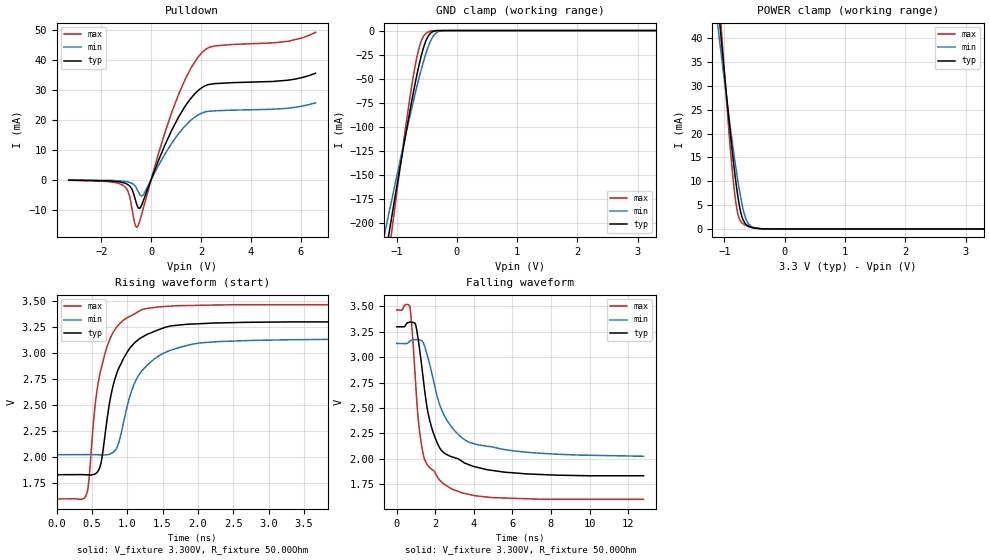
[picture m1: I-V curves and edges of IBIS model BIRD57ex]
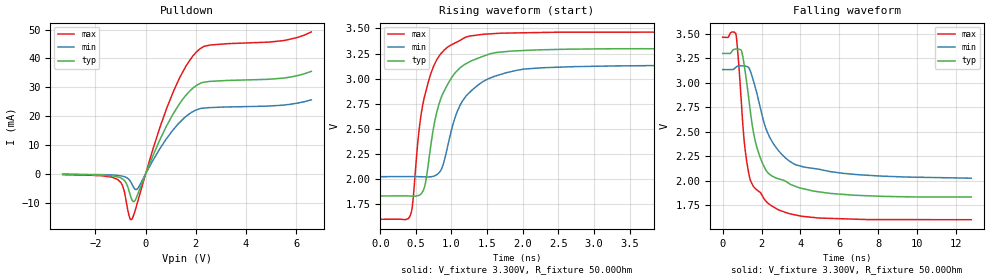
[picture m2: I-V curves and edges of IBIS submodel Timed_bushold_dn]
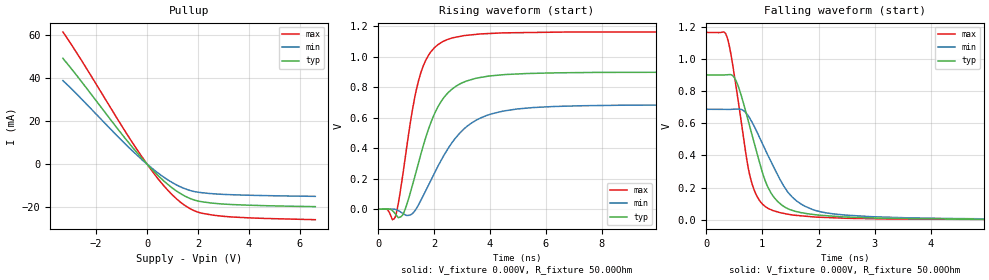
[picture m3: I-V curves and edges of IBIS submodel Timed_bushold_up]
[IBIS Ver]   3.2
[File name]   bird57ex.ibs
[File rev]   0.00
[Date]   12/9/98
[Source]   From silicon level BOGUS SPICE model.
[Notes]   The following information uses the features of BIRD57 to
   describe a FICTICIOUS chip which has an active termintor.
[Disclaimer] This information is only for demonstrating how BIRD57
   works and does not represent any real device in production
   or design.
   WARNING: THIS MODEL HAS NOT BEEN CHECKED USING IBISCHK3.2
   WHICH IS UNDER DEVELOPMENT.  IT MAY CONTAIN SYNTAX ERRORS.
[Copyright]   None - public sample
[Component]   BIRD57ex
[Manufacturer]  Nobody
[Package]
|   typ   min   max
R_pkg   100.00mOhm   NA   NA
L_pkg   8.00nH   NA   NA
C_pkg   5.00pF   NA   NA
[Pin]   signal_name   model_name   R_pin   L_pin   C_pin
1   Vcc   POWER
2   GND   GND
3   Data   BIRD57ex
| Models and submodels in the file (3): BIRD57ex (I/O_open_sink), Timed_bushold_dn (Bus_hold), Timed_bushold_up (Bus_hold)
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[Model]   BIRD57ex
Model_type   I/O_open_sink
Vinl = 800.00mV
Vinh = 2.00V
Vmeas = 1.50V
Cref = 0.00F
|   typ   min   max
C_comp   4.00pF   2.00pF   6.00pF
[Voltage Range]   3.300V   3.135V   3.465V
[Temperature Range]   50.0   100.0   0.0
[Add Submodel]
| name   mode
Timed_bushold_up   All
Timed_bushold_dn   Non-Driving
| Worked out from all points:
|   slope of the pulldown table from 0 to 0.495 V, typ, clamps not added: 47.7 ohm
|   GND clamp passes 1 mA (typ) near -0.39 V on its own axis
|   POWER clamp passes 1 mA (typ) near -0.64 V on its own axis
|   falling waveform, V_fixture 3.300V, R_fixture 50.00Ohm: 20-80 % time 941ps typ, 1.42ns min, 633ps max; typ from 3.3 V to 1.83 V
|   rising waveform, V_fixture 3.300V, R_fixture 50.00Ohm: 20-80 % time 328ps typ, 412ps min, 250ps max; typ from 1.83 V to 3.3 V
[Pulldown]
|   Voltage   I(typ)   I(min)   I(max)
-3.3V     -135.8uA   -78.2uA    -215.1uA
-1.025V   -1.197mA   NA         NA
-785mV    -2.945mA   -1.129mA   NA
-705mV    -4.542mA   NA         NA
-555mV    -8.746mA   NA         NA
-365mV    -8.224mA   NA         NA
825mV     16.45mA    NA         NA
1.46V     25.65mA    NA         NA
2.055V    30.81mA    NA         NA
2.56V     32.06mA    NA         NA
5.47V     33.18mA    NA         NA
6.6V      35.53mA    25.66mA    49.18mA
[GND Clamp]
|   Voltage   I(typ)   I(min)   I(max)
-3.3V     -1.1A      -859.8mA   -1.35A
-1.265V   -264.8mA   NA         -300.4mA
-1.135V   -214.8mA   NA         -235.9mA
-1.075V   -191.9mA   NA         NA
-825mV    -99.88mA   NA         NA
-690mV    -54.59mA   NA         NA
-585mV    -25.13mA   -39.38mA   NA
-520mV    -11.92mA   -25.29mA   NA
-460mV    -4.469mA   NA         NA
-370mV    -529.2uA   NA         NA
-285mV    -44.47uA   NA         NA
3.3V      0A         0A         0A
[POWER Clamp]
|   Voltage   I(typ)   I(min)   I(max)
-3.3V     370mA      287.5mA    500mA
-1.145V   52.63mA    46.39mA    NA
-1.095V   45.64mA    41.06mA    NA
-1.045V   38.76mA    35.79mA    NA
-895mV    19.25mA    NA         15.81mA
-820mV    10.8mA     13.69mA    NA
-775mV    6.621mA    NA         NA
-735mV    3.82mA     NA         NA
-655mV    1.132mA    2.538mA    NA
-575mV    429.4uA    NA         NA
-365mV    19.18uA    NA         NA
3.3V      0A         0A         0A
[Ramp]
R_load = 50.00Ohm
|   typ   min   max
dV/dt_r   540.04mV/1.04ns   411.75mV/1.47ns   698.42mV/705.58ps
dV/dt_f   879.96mV/936.61ps   666.10mV/1.42ns   1.12V/623.48ps
[Falling Waveform]
V_fixture = 3.300V
V_fixture_min = 3.135V
V_fixture_max = 3.465V
R_fixture = 50.00Ohm
|   Time   V(typ)   V(min)   V(max)
0s        3.3V       3.135V     3.465V
670ps     3.346V     NA         NA
970ps     3.324V     NA         NA
1.18ns    3.084V     NA         NA
1.45ns    2.666V     NA         NA
1.78ns    2.326V     NA         NA
2.42ns    2.063V     NA         NA
3.18ns    2.001V     NA         NA
3.96ns    1.926V     NA         NA
12.8ns    1.833V     2.025V     1.601V
[Rising Waveform]
V_fixture = 3.300V
V_fixture_min = 3.135V
V_fixture_max = 3.465V
R_fixture = 50.00Ohm
|   Time   V(typ)   V(min)   V(max)
0s        1.833V     2.025V     1.601V
370ps     1.834V     NA         NA
490ps     1.83V      NA         NA
580ps     1.86V      NA         NA
710ps     2.339V     NA         NA
850ps     2.802V     NA         NA
1.05ns    3.058V     NA         NA
1.28ns    3.178V     NA         NA
2.67ns    3.294V     NA         NA
12.8ns    3.3V       3.135V     3.465V
[Submodel]   Timed_bushold_dn
Submodel_type   Bus_hold
[Submodel Spec]
|   typ   min   max
V_trigger_r   15.00   15.00   15.00
V_trigger_f   1.65   1.50   1.80
Off_delay   5.00ns   3.00ns   7.00ns
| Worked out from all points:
|   slope of the pulldown table from 0 to 0.3 V, typ, clamps not added: 46.2 ohm
|   falling waveform, V_fixture 3.300V, R_fixture 50.00Ohm: 20-80 % time 941ps typ, 1.42ns min, 633ps max; typ from 3.3 V to 1.83 V
|   rising waveform, V_fixture 3.300V, R_fixture 50.00Ohm: 20-80 % time 328ps typ, 412ps min, 250ps max; typ from 1.83 V to 3.3 V
[Pulldown]
|   Voltage   I(typ)   I(min)   I(max)
-3.3V     -135.8uA   -78.2uA    -215.1uA
-1.025V   -1.197mA   NA         NA
-785mV    -2.945mA   -1.129mA   NA
-705mV    -4.542mA   NA         NA
-555mV    -8.746mA   NA         NA
-365mV    -8.224mA   NA         NA
825mV     16.45mA    NA         NA
1.46V     25.65mA    NA         NA
2.055V    30.81mA    NA         NA
2.56V     32.06mA    NA         NA
5.47V     33.18mA    NA         NA
6.6V      35.53mA    25.66mA    49.18mA
[Ramp]
R_load = 50.00Ohm
|   typ   min   max
dV/dt_r   540.04mV/1.04ns   411.75mV/1.47ns   698.42mV/705.58ps
dV/dt_f   879.96mV/936.61ps   666.10mV/1.42ns   1.12V/623.48ps
[Falling Waveform]
V_fixture = 3.300V
V_fixture_min = 3.135V
V_fixture_max = 3.465V
R_fixture = 50.00Ohm
|   Time   V(typ)   V(min)   V(max)
0s        3.3V       3.135V     3.465V
670ps     3.346V     NA         NA
970ps     3.324V     NA         NA
1.18ns    3.084V     NA         NA
1.45ns    2.666V     NA         NA
1.78ns    2.326V     NA         NA
2.42ns    2.063V     NA         NA
3.18ns    2.001V     NA         NA
3.96ns    1.926V     NA         NA
12.8ns    1.833V     2.025V     1.601V
[Rising Waveform]
V_fixture = 3.300V
V_fixture_min = 3.135V
V_fixture_max = 3.465V
R_fixture = 50.00Ohm
|   Time   V(typ)   V(min)   V(max)
0s        1.833V     2.025V     1.601V
370ps     1.834V     NA         NA
490ps     1.83V      NA         NA
580ps     1.86V      NA         NA
710ps     2.339V     NA         NA
850ps     2.802V     NA         NA
1.05ns    3.058V     NA         NA
1.28ns    3.178V     NA         NA
2.67ns    3.294V     NA         NA
12.8ns    3.3V       3.135V     3.465V
[Submodel]   Timed_bushold_up
Submodel_type   Bus_hold
[Submodel Spec]
|   typ   min   max
V_trigger_r   1.65   1.50   1.80
V_trigger_f   -10.00   -10.00   -10.00
Off_delay   5.00ns   3.00ns   7.00ns
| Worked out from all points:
|   slope of the pullup table from 0 to 0.3 V, typ, clamps not added: 79.2 ohm
|   rising waveform, V_fixture 0.000V, R_fixture 50.00Ohm: 20-80 % time 1.04ns typ, 1.47ns min, 707ps max; typ from 0 V to 0.9 V
|   falling waveform, V_fixture 0.000V, R_fixture 50.00Ohm: 20-80 % time 466ps typ, 643ps min, 322ps max; typ from 0.9 V to 0 V
[Pullup]
|   Voltage   I(typ)   I(min)   I(max)
-3.3V     49.3mA     38.93mA    61.61mA
-2.685V   40.22mA    NA         NA
-905mV    12.69mA    NA         NA
0V        19.8nA     -62.62nA   30.91nA
675mV     -8.054mA   NA         NA
1.045V    -11.64mA   NA         NA
1.395V    -14.36mA   NA         NA
1.735V    -16.29mA   NA         NA
2.055V    -17.39mA   NA         NA
2.875V    -18.57mA   NA         NA
3.89V     -19.15mA   NA         NA
6.6V      -19.87mA   -15.07mA   -25.95mA
[Ramp]
R_load = 50.00Ohm
|   typ   min   max
dV/dt_r   540.04mV/1.04ns   411.75mV/1.47ns   698.42mV/705.58ps
dV/dt_f   879.96mV/936.61ps   666.10mV/1.42ns   1.12V/623.48ps
[Rising Waveform]
V_fixture = 0.000V
V_fixture_min = 0.000V
V_fixture_max = 0.000V
R_fixture = 50.00Ohm
|   Time   V(typ)   V(min)   V(max)
0s        0V         0V         0V
560ps     -18.13mV   NA         NA
910ps     -25.05mV   NA         NA
1.28ns    193.5mV    -17.59mV   NA
1.55ns    377.6mV    NA         NA
1.96ns    604.2mV    NA         NA
2.38ns    740.6mV    NA         NA
3.14ns    840.8mV    NA         NA
4.54ns    884.4mV    NA         NA
12.8ns    900.1mV    686.2mV    1.164V
[Falling Waveform]
V_fixture = 0.000V
V_fixture_min = 0.000V
V_fixture_max = 0.000V
R_fixture = 50.00Ohm
|   Time   V(typ)   V(min)   V(max)
0s        900.1mV    686.2mV    1.164V
320ps     899.6mV    NA         NA
520ps     872.4mV    NA         NA
680ps     704.5mV    NA         NA
890ps     432.7mV    NA         NA
1.08ns    217.1mV    NA         NA
1.28ns    110.8mV    NA         NA
1.68ns    44.43mV    NA         NA
2.42ns    17.64mV    NA         NA
12.8ns    0V         0V         0V
